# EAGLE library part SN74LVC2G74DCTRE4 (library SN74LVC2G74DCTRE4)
Flip Flops Single Pos Edge Trig Source: Datasheet
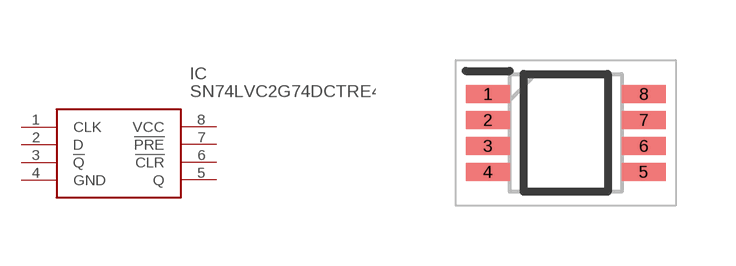
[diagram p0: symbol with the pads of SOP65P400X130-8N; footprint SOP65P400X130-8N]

Designator prefix IC

## SN74LVC2G74DCTRE4 (Description: Flip Flops Single Pos Edge Trig; Height: 1.3mm; Manufacturer_Name: Texas Instruments; Manufacturer_Part_Number: SN74LVC2G74DCTRE4; Mouser_Part_Number: 595-SN74LVC2G74DCTE4; Mouser_Price-Stock: https://www.mouser.co.uk/ProductDetail/Texas-Instruments/SN74LVC2G74DCTRE4?qs=0smPjiIwnfIl%2Fv02vJdCHg%3D%3D)  [SOP65P400X130-8N]
1  CLK  in
2  D  in
3  !Q  out
4  GND  pwr
5  Q  out
6  !CLR  in
7  !PRE  in
8  VCC  pwr

## Footprint SOP65P400X130-8N (pad centres in mm)
DCT (R-PDSO-G8)
smd 1.1 x 0.45: 1 -1.95,0.975; 2 -1.95,0.325; 3 -1.95,-0.325; 4 -1.95,-0.975; 5 1.95,-0.975; 6 1.95,-0.325; 7 1.95,0.325; 8 1.95,0.975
